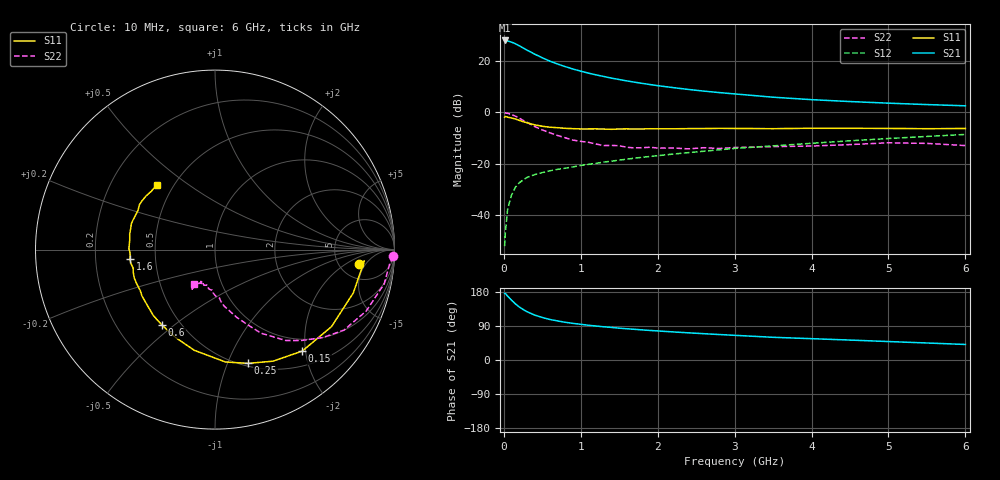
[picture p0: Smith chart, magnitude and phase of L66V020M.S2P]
!  INFINEON TECHNOLOGIES Small Signal Semiconductors
! BFR380L3 , Si-NPN RF-Transistor in TSLP-3-1
!  Vce=6 V,  Ic=20 mA
! Common Emitter S-Parameters:  07. March 2005
#  GHz  S  MA  R  50
! f  S11  S21  S12  S22
! GHz  Mag  Ang  Mag  Ang  Mag  Ang  Mag  Ang
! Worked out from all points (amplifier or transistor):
!   36 points, 10 MHz to 6 GHz, reference 50 ohm
!   highest |S21| = 28.2 dB at 10 MHz (marker M1)
!   |S21| within 3 dB of that: start of sweep to 255.4 MHz
!   unconditionally stable (mu >= 1): 2.319 GHz to 4.712 GHz
!   at 250 MHz: K = 0.30, MSG = 25.9 dB, |S12| = -26.4 dB
!   at 1.4 GHz: K = 0.90, MSG = 16.3 dB, |S12| = -19.1 dB
!   at 6 GHz: K = 0.97, MSG = 5.6 dB, |S12| = -8.6 dB
!   S11 on the Smith chart (normalised r, x): 10 MHz: 7.69, -3.62; 150 MHz: 0.76, -1.94; 250 MHz: 0.53, -1.19; 600 MHz: 0.40, -0.45; 1.6 GHz: 0.36, -0.05; 6 GHz: 0.41, +0.38
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0.01  0.8081 -5.8  25.75 175.6  0.0024 70.6  0.9938 -2.2
0.02  0.8345 -4.3  25.49 175.4  0.0045 86.9  0.9764 -4.7
0.05  0.8074 -17.4  25.18 168.4  0.0129 80.5  0.962 -11.4
0.1  0.7781 -33.5  23.85 157.9  0.024 74.0  0.9095 -22.1
0.15  0.7457 -49.3  22.19 148.2  0.0342 67.0  0.8469 -32.0
0.2  0.7008 -62.5  20.25 140.0  0.0418 63.6  0.7754 -39.2
0.25  0.6601 -73.8  18.43 133.5  0.0476 57.7  0.6992 -46.4
0.3  0.6289 -84.7  16.7 127.5  0.0532 55.8  0.6418 -52.1
0.4  0.5728 -101.6  13.92 118.6  0.0605 51.8  0.5312 -61.2
0.5  0.5365 -114.3  11.78 112.2  0.0665 50.7  0.4544 -66.7
0.6  0.5135 -125.3  10.12 106.9  0.072 50.5  0.3984 -72.0
0.7  0.503 -133.1  8.881 103.0  0.077 51.2  0.3532 -76.4
0.8  0.4882 -140.7  7.899 99.5  0.081 51.6  0.3188 -80.8
0.9  0.482 -147.6  7.082 96.6  0.0857 52.6  0.2873 -83.8
1.1  0.4759 -156.3  5.903 91.7  0.0963 54.3  0.2601 -89.0
1.4  0.4678 -167.3  4.709 86.0  0.111 56.3  0.2262 -95.3
1.6  0.4769 -174.0  4.151 82.4  0.1217 57.4  0.2077 -102.5
2.2  0.4782 173.4  3.069 74.1  0.153 59.7  0.2013 -108.1
3.5  0.4816 153.1  1.991 59.9  0.2215 60.6  0.2143 -117.6
4.5  0.4889 146.1  1.636 52.6  0.2785 60.5  0.2348 -119.4
5.5  0.4811 137.6  1.427 44.9  0.3389 58.0  0.2476 -120.2
6  0.4851 132.1  1.35 41.0  0.371 56.2  0.2243 -120.8
